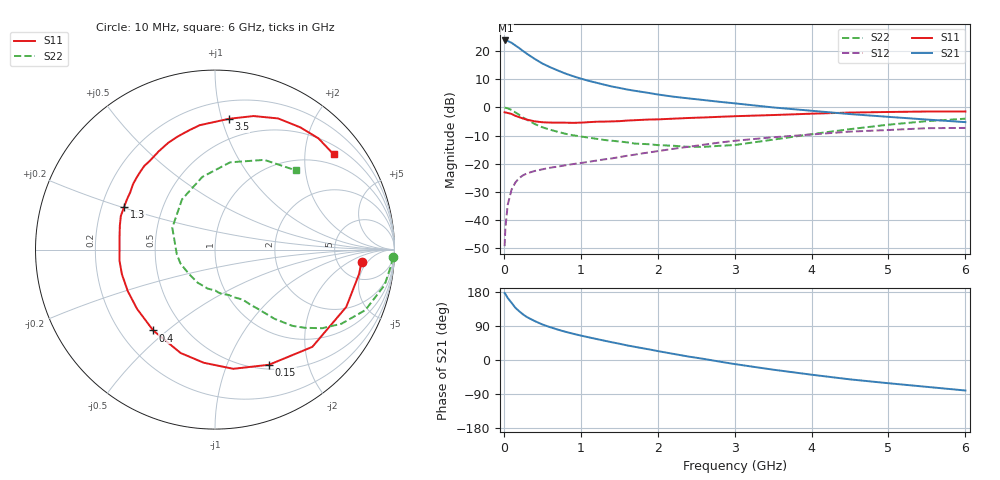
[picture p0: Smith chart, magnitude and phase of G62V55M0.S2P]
! SIEMENS Small Signal Semiconductors
! BFG193
! Si NPN RF Bipolar Junction Transistor in SOT223
! VCE = 2.5 V  IC = 5 mA
! Common Emitter S-Parameters:  August  1996
# GHz  S  MA  R  50
!  f  S11  S21  S12  S22
! GHz  MAG  ANG  MAG  ANG  MAG  ANG  MAG  ANG
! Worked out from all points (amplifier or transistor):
!   36 points, 10 MHz to 6 GHz, reference 50 ohm
!   highest |S21| = 23.8 dB at 20 MHz (marker M1)
!   |S21| within 3 dB of that: start of sweep to 213.6 MHz
!   unconditionally stable (mu >= 1): 1.096 GHz to 2.624 GHz
!   at 250 MHz: K = 0.34, MSG = 22.1 dB, |S12| = -24.1 dB
!   at 1.4 GHz: K = 1.09, MAG = 11.0 dB, |S12| = -18.1 dB
!   at 6 GHz: K = 0.90, MSG = 1.0 dB, |S12| = -7.3 dB
!   S11 on the Smith chart (normalised r, x): 10 MHz: 8.63, -3.53; 150 MHz: 0.55, -1.42; 400 MHz: 0.34, -0.45; 1.3 GHz: 0.30, +0.20; 3.5 GHz: 0.33, +1.05; 6 GHz: 0.71, +2.68
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0.01  0.8196 -4.7  15.54 176.7  0.0034 89.5  0.9905 -2.4
0.02  0.8142 -9.6  15.57 174.3  0.0071 84.4  0.9866 -4.7
0.05  0.7981 -23.6  15.23 163.8  0.0184 77.9  0.9655 -11.8
0.1  0.7666 -45.0  14.15 151.1  0.0344 68.2  0.903 -21.9
0.15  0.7086 -64.9  12.68 137.8  0.0462 58.9  0.8166 -30.4
0.2  0.6719 -81.3  11.39 128.6  0.0555 52.9  0.7401 -36.3
0.25  0.6335 -95.7  10.1 120.2  0.0621 47.9  0.6626 -41.1
0.3  0.6071 -108.4  9.02 113.3  0.067 44.9  0.6049 -44.6
0.4  0.567 -127.4  7.328 102.9  0.074 40.5  0.5087 -49.3
0.5  0.5456 -142.8  6.063 93.8  0.0792 37.8  0.4443 -52.1
0.6  0.5382 -154.5  5.215 86.7  0.0845 37.1  0.4026 -54.4
0.7  0.5366 -165.1  4.558 80.3  0.0885 36.9  0.3685 -57.0
0.9  0.5318 179.0  3.601 69.3  0.0983 36.9  0.3196 -60.9
1.1  0.5465 166.0  2.984 60.0  0.1077 37.4  0.2904 -67.1
1.3  0.5592 155.0  2.554 51.3  0.1188 37.3  0.2645 -73.0
1.6  0.5844 141.4  2.089 38.6  0.1378 36.3  0.2394 -85.6
2.2  0.6312 119.7  1.557 16.3  0.1835 31.1  0.2083 -117.4
2.8  0.6809 102.0  1.262 -4.1  0.2369 21.9  0.2074 -158.7
3.5  0.7326 84.0  1.001 -25.5  0.2948 6.8  0.2673 152.9
4.5  0.811 64.3  0.762 -51.1  0.3715 -13.6  0.4111 99.9
5.5  0.8463 47.1  0.609 -70.9  0.4274 -39.0  0.5705 61.2
6  0.8478 38.7  0.548 -80.5  0.4324 -53.3  0.6312 44.3
